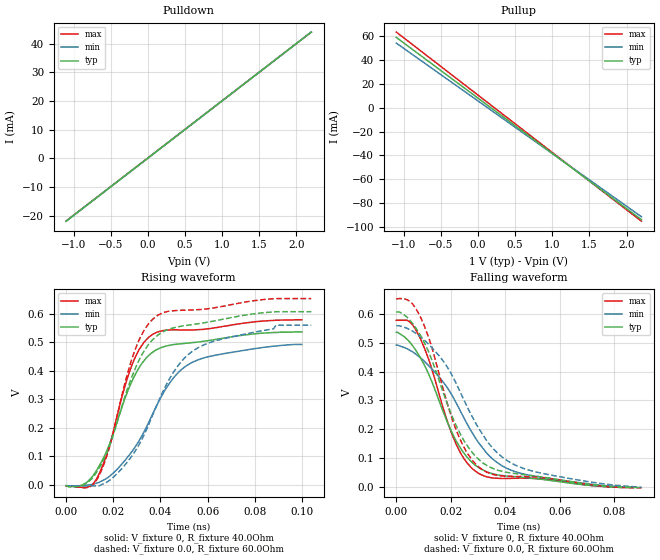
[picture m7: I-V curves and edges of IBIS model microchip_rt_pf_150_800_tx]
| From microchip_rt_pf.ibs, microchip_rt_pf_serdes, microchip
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[Model]   microchip_rt_pf_150_800_tx
Model_type   Output
Polarity   Non-Inverting
Enable   Active-High
Vmeas = 0.5
|   typ   min   max
C_comp   0.407p  0.407p  0.407p
[Voltage Range]   1.0  0.9  1.1
[Temperature Range]   27  27  27
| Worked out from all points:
|   slope of the pulldown table from 0 to 0.15 V, typ, clamps not added: 50.1 ohm
|   slope of the pullup table from 0 to 0.15 V, typ, clamps not added: 21.6 ohm
|   rising waveform, V_fixture 0, R_fixture 40.0Ohm: 20-80 % time 15.9ps typ, 21.6ps min, 12.8ps max; typ from -0.003 V to 0.537 V
|   rising waveform, V_fixture 0.0, R_fixture 60.0Ohm: 20-80 % time 16.8ps typ, 22ps min, 13.5ps max; typ from -0.003 V to 0.608 V
|   falling waveform, V_fixture 0, R_fixture 40.0Ohm: 20-80 % time 15.7ps typ, 20.6ps min, 12.7ps max; typ from 0.538 V to -0.002 V
|   falling waveform, V_fixture 0.0, R_fixture 60.0Ohm: 20-80 % time 16.8ps typ, 21.6ps min, 13.6ps max; typ from 0.608 V to -0.004 V
[Pullup]
|   X   TYP   MIN   MAX
-1.1V     59.06mA    54.28mA    63.55mA
1.01V     -38.83mA   -38.99mA   -38.07mA
1.066V    -41.43mA   -41.47mA   -40.77mA
2.2V      -94.02mA   -91.58mA   -95.36mA
[Pulldown]
|   X   TYP   MIN   MAX
-1.1V     -21.83mA   -21.86mA   -21.76mA
1.01V     20.27mA    20.26mA    20.29mA
1.089V    21.83mA    21.82mA    21.86mA
2.2V      44mA       44mA       44mA
[Ramp]
R_load = 50.0Ohm
|   typ   min   max
dV/dt_r   3.24E-1V/1.59E-2ns   2.98E-1V/2.16E-2ns   3.50E-1V/1.28E-2ns
dV/dt_f   3.24E-1V/1.57E-2ns   2.97E-1V/2.07E-2ns   3.50E-1V/1.27E-2ns
[Rising Waveform]
V_fixture   = 0
V_fixture_min = 0
V_fixture_max = 0
R_fixture   = 40.0Ohm
|   Time   V(typ)   V(min)   V(max)
0s        -3mV       -3mV       -4mV
7ps       -26.95uV   -3mV       -9.003mV
13ps      51.43mV    6.039mV    21.44mV
18ps      134.4mV    27.16mV    127.1mV
28ps      365.2mV    117.7mV    422.4mV
31ps      412.2mV    155.5mV    475.6mV
36ps      461.4mV    236.3mV    524.3mV
45ps      491.9mV    369.5mV    544.4mV
54ps      500mV      432mV      543.9mV
100ps     537mV      493mV      579.5mV
[Rising Waveform]
V_fixture   = 0.0
V_fixture_min = 0.0
V_fixture_max = 0.0
R_fixture   = 60.0Ohm
|   Time   V(typ)   V(min)   V(max)
0s        -3mV       -3.5mV     -4.5mV
7ps       -2.517mV   -3.5mV     -10.03mV
14ps      58.77mV    -3.5mV     32.63mV
18ps      127.2mV    13.32mV    120.2mV
29ps      401.5mV    114.5mV    468.4mV
38ps      519.3mV    270.5mV    589.9mV
47ps      554.1mV    413.1mV    612.2mV
57ps      567.2mV    486.3mV    615.7mV
89ps      608mV      560.5mV    654mV
104ps     608mV      560.5mV    654mV
[Falling Waveform]
V_fixture   = 0
V_fixture_min = 0
V_fixture_max = 0
R_fixture   = 40.0Ohm
|   Time   V(typ)   V(min)   V(max)
0s        537.5mV    493mV      579.5mV
4ps       512.5mV    480.3mV    579.5mV
8ps       462.4mV    455.3mV    531.7mV
12ps      389.3mV    420.3mV    440.2mV
21ps      177.2mV    309.2mV    169.4mV
25ps      114.5mV    236.2mV    95.31mV
29ps      74.29mV    170.3mV    53.88mV
36ps      43.15mV    91.19mV    29.39mV
45ps      33.11mV    47.93mV    29.38mV
87ps      -2.5mV     -1.5mV     -3.5mV
[Falling Waveform]
V_fixture   = 0.0
V_fixture_min = 0.0
V_fixture_max = 0.0
R_fixture   = 60.0Ohm
|   Time   V(typ)   V(min)   V(max)
0s        608.5mV    560.5mV    654mV
5ps       579.4mV    546.3mV    645.1mV
9ps       525.1mV    520.8mV    588.1mV
16ps      361.7mV    452.8mV    382.8mV
22ps      212.1mV    359.1mV    197.2mV
26ps      143.1mV    278.6mV    117.1mV
31ps      88.68mV    191.9mV    62.96mV
39ps      52.39mV    101.8mV    36.63mV
47ps      41.3mV     62.12mV    35.14mV
90ps      -3.5mV     -2mV       -4.5mV
[Algorithmic Model]
Executable Linux_gcc5.4_64   MPF300T-TX_LX64.so   MPF300T-TX-R150_800.ami
Executable Windows_cl18.00.40629_64 MPF300T-TX_WIN64.dll  MPF300T-TX-R150_800.ami
Executable Windows_cl18.00.40629_32 MPF300T-TX_WIN32.dll  MPF300T-TX-R150_800.ami
[End Algorithmic Model]
